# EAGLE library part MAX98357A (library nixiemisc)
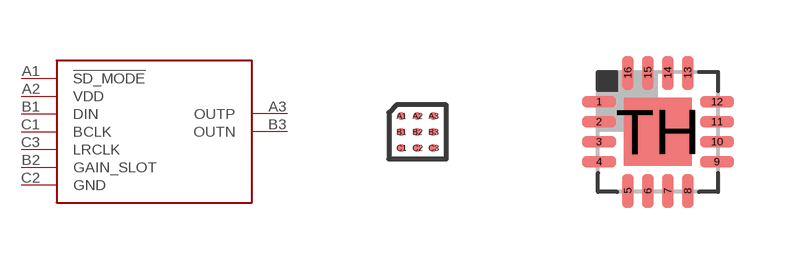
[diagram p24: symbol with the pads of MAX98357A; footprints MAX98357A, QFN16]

Designator prefix U

## MAX98357A  [MAX98357A]
A1  !SD_MODE
A2  VDD
A3  OUTP
B1  DIN
B2  GAIN_SLOT
B3  OUTN
C1  BCLK
C2  GND
C3  LRCLK

## MAX98357AQFN  [QFN16]
1  DIN
2  GAIN_SLOT
3  GND
4  !SD_MODE
7  VDD
8  VDD
9  OUTP
10  OUTN
11  GND
14  LRCLK
15  GND
16  BCLK
TH  GND

## Footprint MAX98357A (pad centres in mm)
smd 0.2 x 0.2: A1 -0.4,0.4; A2 0,0.4; A3 0.4,0.4; B1 -0.4,0; B2 0,0; B3 0.4,0; C1 -0.4,-0.4; C2 0,-0.4; C3 0.4,-0.4

## Footprint QFN16 (pad centres in mm)
RTE (S-PQFP-N16) 3x3 mm Source: www.ti.com .. tpa6132a2 direct path stereo $.65.pdf
smd 0.85 x 0.28: 1 -1.475,0.75; 2 -1.475,0.25; 3 -1.475,-0.25; 4 -1.475,-0.75; 9 1.475,-0.75; 10 1.475,-0.25; 11 1.475,0.25; 12 1.475,0.75
smd 0.28 x 0.85: 5 -0.75,-1.475; 6 -0.25,-1.475; 7 0.25,-1.475; 8 0.75,-1.475; 13 0.75,1.475; 14 0.25,1.475; 15 -0.25,1.475; 16 -0.75,1.475
smd 1.7 x 1.7: TH 0,0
